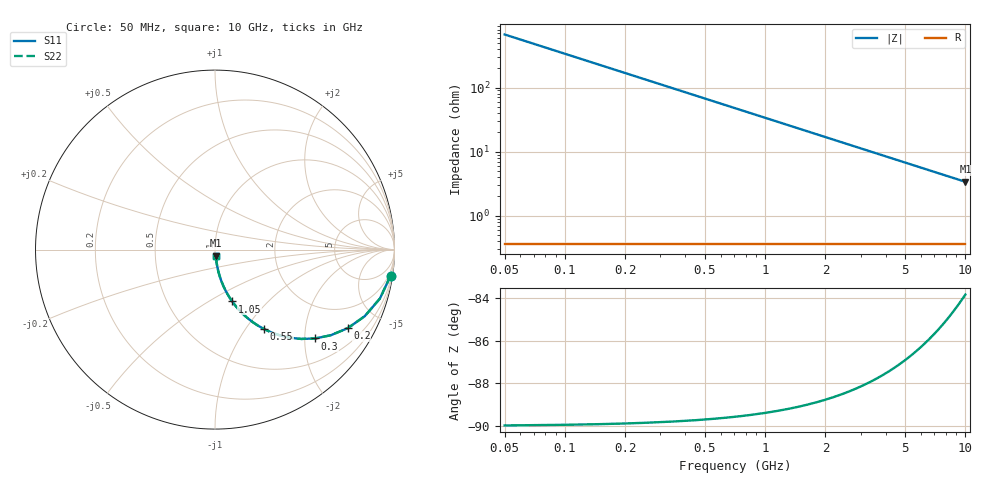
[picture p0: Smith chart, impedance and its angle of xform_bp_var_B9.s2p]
! Created Wed Dec 13 22:21:55 2017
# ghz S ma R 50
! 2 Port Network Data from SP1.SP block
! freq  magS11  angS11  magS21  angS21  magS12  angS12  magS22  angS22
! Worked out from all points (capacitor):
!   200 points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, 50 MHz to 10 GHz, reference 50 ohm
!   read as one part in series: C = 4.73 pF near 100 MHz
!   lowest |Z| = 3.39 ohm at 10 GHz (marker M1)
!   S11 on the Smith chart (normalised r, x): 50 MHz: 1, -13; 200 MHz: 1.01, -3.37; 300 MHz: 1.01, -2.24; 550 MHz: 1.01, -1.22; 1.05 GHz: 1.01, -0.64; 10 GHz: 1.01, -0.07
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0.05  0.9891 -8.4  0.1469 81.5  0.1469 81.5  0.9891 -8.4
0.1  0.9583 -16.5  0.2846 73.4  0.2846 73.4  0.9583 -16.5
0.15  0.9129 -24.0  0.4067 65.9  0.4067 65.9  0.9129 -24.0
0.2  0.859 -30.7  0.5102 59.2  0.5102 59.2  0.859 -30.7
0.25  0.8019 -36.5  0.5953 53.3  0.5953 53.3  0.8019 -36.5
0.3  0.7455 -41.6  0.6641 48.2  0.6641 48.2  0.7455 -41.6
0.4  0.6427 -49.8  0.7634 40.0  0.7634 40.0  0.6427 -49.8
0.45  0.5977 -53.0  0.7988 36.7  0.7988 36.7  0.5977 -53.0
0.55  0.5208 -58.3  0.8506 31.4  0.8506 31.4  0.5208 -58.3
0.65  0.4587 -62.3  0.8854 27.3  0.8854 27.3  0.4587 -62.3
0.75  0.4084 -65.4  0.9095 24.1  0.9095 24.1  0.4084 -65.4
0.9  0.3493 -69.0  0.9336 20.4  0.9336 20.4  0.3493 -69.0
1.05  0.3044 -71.6  0.9491 17.7  0.9491 17.7  0.3044 -71.6
1.4  0.2331 -75.7  0.9689 13.5  0.9689 13.5  0.2331 -75.7
1.75  0.1883 -78.1  0.9786 10.9  0.9786 10.9  0.1883 -78.1
2.5  0.1331 -80.8  0.9875 7.6  0.9875 7.6  0.1331 -80.8
3.4  0.09827 -82.3  0.9916 5.6  0.9916 5.6  0.09827 -82.3
4.15  0.08066 -82.8  0.9931 4.6  0.9931 4.6  0.08066 -82.8
5.05  0.06639 -83.1  0.9942 3.8  0.9942 3.8  0.06639 -83.1
6.7  0.05014 -83.0  0.9951 2.9  0.9951 2.9  0.05014 -83.0
8.35  0.04031 -82.6  0.9956 2.3  0.9956 2.3  0.04031 -82.6
10  0.03373 -81.9  0.9958 1.9  0.9958 1.9  0.03373 -81.9
